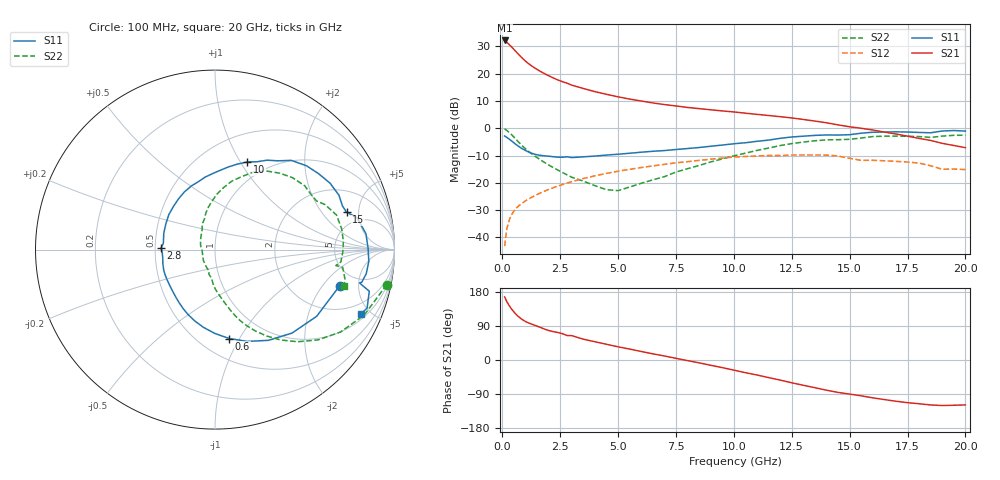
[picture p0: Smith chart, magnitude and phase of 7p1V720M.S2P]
! Infineon Technologies  Discrete & RF Semiconductors
! bfp620
! VCE =  1.7 V,  IC =  20 mA
! Common Emitter S-Parameters:  Sep 2002
# GHz  S  MA  R  50
!  f  S11  S21  S12  S22
! GHz  MAG  ANG  MAG  ANG  MAG  ANG  MAG  ANG
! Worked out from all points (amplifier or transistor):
!   59 points, 100 MHz to 20 GHz, reference 50 ohm
!   highest |S21| = 32.2 dB at 100 MHz (marker M1)
!   |S21| within 3 dB of that: start of sweep to 472.1 MHz
!   unconditionally stable (mu >= 1): 3.431 GHz to 9.942 GHz; 17.15 GHz to end of sweep
!   at 1 GHz: K = 0.68, MSG = 25.6 dB, |S12| = -26.6 dB
!   at 5.5 GHz: K = 1.04, MAG = 11.7 dB, |S12| = -15.1 dB
!   at 20 GHz: K = 1.31, MAG = 0.7 dB, |S12| = -15.1 dB
!   S11 on the Smith chart (normalised r, x): 100 MHz: 3.54, -3.01; 600 MHz: 0.68, -0.91; 2.8 GHz: 0.54, +0.01; 10 GHz: 0.80, +1.07; 15 GHz: 3.65, +3.63; 20 GHz: 1.28, -4.35
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0.1  0.7228 -16.3  40.66 166.6  0.0069 81.5  0.9769 -11.5
0.2  0.6774 -33.3  37.38 153.6  0.0146 74.0  0.9079 -23.7
0.3  0.6329 -47.3  34.21 143.2  0.0208 69.4  0.8366 -33.3
0.4  0.5867 -59.5  31.03 134.4  0.026 65.7  0.7626 -41.3
0.5  0.542 -70.7  27.96 126.9  0.0303 62.8  0.6897 -48.1
0.6  0.5017 -80.9  25.14 120.2  0.0341 60.6  0.6214 -54.1
0.7  0.4669 -90.2  22.63 114.4  0.0375 58.9  0.56 -59.2
0.9  0.4126 -106.0  18.61 105.2  0.0437 56.7  0.4602 -67.3
1  0.3914 -112.6  17.04 101.7  0.0467 56.1  0.4209 -70.4
1.2  0.3577 -123.8  14.57 96.2  0.0523 55.1  0.3583 -75.0
1.5  0.3265 -138.1  11.99 89.4  0.0609 54.0  0.2903 -80.7
1.9  0.3103 -154.7  9.643 79.9  0.0725 52.1  0.2255 -88.7
2.8  0.3001 178.4  6.696 64.5  0.0991 46.6  0.1398 -104.3
3.5  0.2997 162.2  5.357 54.9  0.1199 41.2  0.1074 -117.1
5  0.3342 133.7  3.768 34.8  0.163 28.3  0.072 -176.3
7  0.3901 103.5  2.719 10.6  0.218 9.9  0.1297 123.6
10  0.5197 69.9  1.991 -26.7  0.2964 -22.2  0.3119 87.6
10.5  0.5427 64.4  1.89 -33.5  0.3041 -28.7  0.3495 82.0
13.5  0.7401 30.0  1.355 -73.1  0.323 -64.2  0.5892 42.8
15  0.7619 15.9  1.064 -90.0  0.2817 -85.2  0.6273 25.6
17  0.8595 -4.4  0.786 -108.8  0.2473 -95.8  0.7168 3.7
20  0.8877 -24.0  0.441 -118.6  0.1749 -106.3  0.7452 -15.6
